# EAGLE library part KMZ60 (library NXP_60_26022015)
Angle sensor with integrated amplifier The MagnetoResistive (MR) sensor with integrated amplifier is designed for angular control applications and BrushLess DC (BLDC) motors with even-numbered pole pairs. It consists of two microchips within one package, an angle sensor and an amplifier Integrated Circuit (IC). The circuit delivers cosine and sine output signals related to the angle of a rotating magnetic field. The output voltage range is ratiometric related to the supply voltage. The Temperature Coefficient (TC) of the sensor amplitude can be compensated. A ratiometric output voltage linear to the temperature is delivered. A Power-down mode is implemented. AAL Eindhoven MK
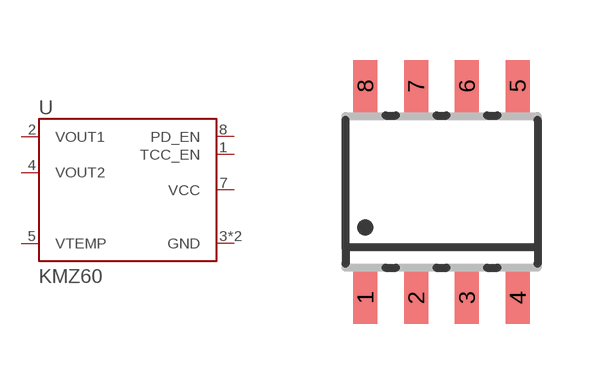
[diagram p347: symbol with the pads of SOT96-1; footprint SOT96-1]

Designator prefix U

## KMZ60  [SOT96-1]
1  TCC_EN  in
2  VOUT1  out
3  GND  pwr
4  VOUT2
5  VTEMP
6  GND  pwr
7  VCC
8  PD_EN  in

## Footprint SOT96-1 (pad centres in mm)
SOT96-1 SO8: plastic small outline package; 8 leads; body width 3.9 mm JEDEC: MS-012 IEC: 076E03
smd 0.6 x 1.3: 1 -1.905,-2.65; 2 -0.635,-2.65; 3 0.635,-2.65; 4 1.905,-2.65; 5 1.905,2.65; 6 0.635,2.65; 7 -0.635,2.65; 8 -1.905,2.65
